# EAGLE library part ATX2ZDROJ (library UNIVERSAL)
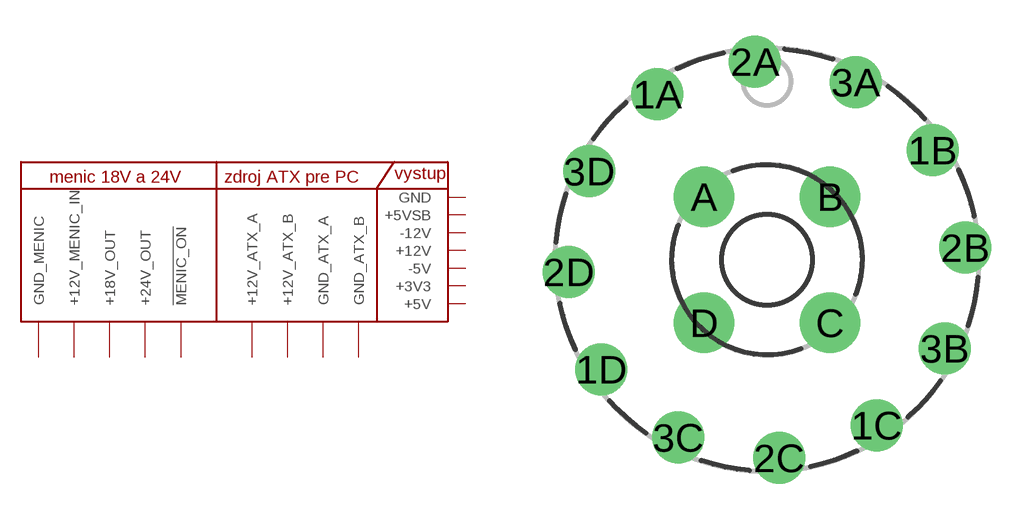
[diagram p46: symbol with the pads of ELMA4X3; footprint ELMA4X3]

Designator prefix Z

## ATX2ZDROJ  [ELMA4X3]
1A  !MENIC_ON
1B  +3V3
1C  +5V
1D  +5VSB
2A  +12V
2B  +12V_ATX_A
2C  +12V_ATX_B
2D  +12V_MENIC_IN
3A  +18V_OUT
3B  +24V_OUT
3C  -5V
3D  -12V
A  GND
B  GND_ATX_A
C  GND_ATX_B
D  GND_MENIC

## Footprint ELMA4X3 (pad centres in mm)
drill 1.3 pad 2.184: 1A -4.609,6.963; 1B 6.963,4.609; 1C 4.609,-6.963; 1D -6.963,-4.609; 2A -0.51,8.334; 2B 8.334,0.51; 2C 0.51,-8.334; 2D -8.334,-0.51; 3A 3.726,7.473; 3B 7.473,-3.726; 3C -3.726,-7.473; 3D -7.473,3.726
drill 1.5 pad 2.54: A -2.652,2.652; B 2.652,2.652; C 2.652,-2.652; D -2.652,-2.652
